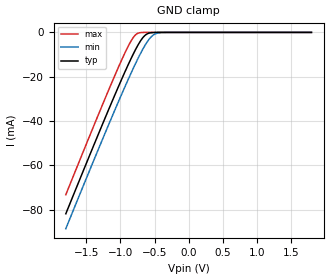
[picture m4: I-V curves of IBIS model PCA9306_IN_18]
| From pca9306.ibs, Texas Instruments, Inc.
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[Model]   PCA9306_IN_18
Model_type  Input
Vinl=0.6
Vinh=1.95
| variable   typ   min   max
C_comp   5.86pF   4.79pF   7.43pF
[Temperature Range]   40   100   -40
| Ambient temperature   25   85   -40
[Voltage range]   1.8   1.65   1.95
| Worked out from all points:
|   GND clamp passes 1 mA (typ) near -0.62 V on its own axis
[GND Clamp]
| PCA9306_IN_18
|   Voltage   I(typ)   I(min)   I(max)
-1.8V     -81.79mA   -88.5mA    -73.19mA
-1.17V    -34.63mA   -41.45mA   -25.82mA
-990mV    -21.72mA   -28.49mA   -13.02mA
-870mV    -13.52mA   -20.14mA   -5.318mA
-820mV    -10.3mA    -16.78mA   -2.695mA
-775mV    -7.564mA   -13.84mA   -1.024mA
-675mV    -2.531mA   -7.765mA   -29.79uA
-610mV    -711.8uA   -4.402mA   -2.004uA
-525mV    -70.21uA   -1.354mA   -57.44nA
-455mV    -8.281uA   -320.7uA   -3.133nA
-345mV    -270.4nA   -21.14uA   -35.62pA
1.8V      36.2pA     2.812nA    28.26pA
